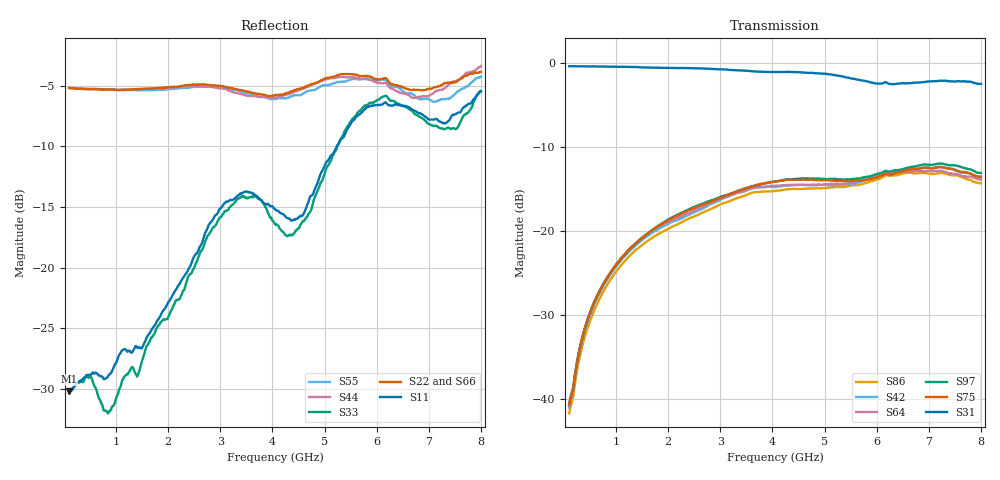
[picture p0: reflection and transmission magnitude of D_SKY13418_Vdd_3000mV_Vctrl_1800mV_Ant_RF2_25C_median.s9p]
# GHz S DB R 50
! THRU S21 mag phase subtraction.
! HALF_THRU
! EN33-165-011-v1_HALF_THRU_1 EN33-165-011-v1_HALF_THRU_2 EN33-165-011-v1_HALF_THRU_3 EN33-165-011-v1_HALF_THRU_4 EN33-165-011-v1_HALF_THRU_5 EN33-165-011-v1_HALF_THRU_6 EN33-165-011-v1_HALF_THRU_7 EN33-165-011-v1_HALF_THRU_8 EN33-165-011-v1_HALF_THRU_9
! THRU Ports: 1 2
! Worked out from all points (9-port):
!   801 points, 100 MHz to 8 GHz, reference 50 ohm
!   strongest paths, dB at 100 MHz, 2.075 GHz, 4.05 GHz, 6.025 GHz, 8 GHz:
!     S31: -0.4, -0.6, -1.0, -2.4, -2.5
!     S75: -40.7, -18.4, -14.1, -13.5, -13.5
!     S97: -40.5, -18.4, -14.1, -13.1, -13.1
!     S64: -40.8, -18.7, -14.6, -13.4, -13.9
!     S42: -41.0, -18.9, -14.7, -13.5, -13.7
!     S86: -41.7, -19.5, -15.2, -13.8, -14.3
!   lowest |S11| = -30.2 dB at 100 MHz (marker M1), VSWR 1.06, Z = 53.2 + j0.407 ohm
!   |S11| at or under -10 dB: start of sweep to 5.235 GHz
